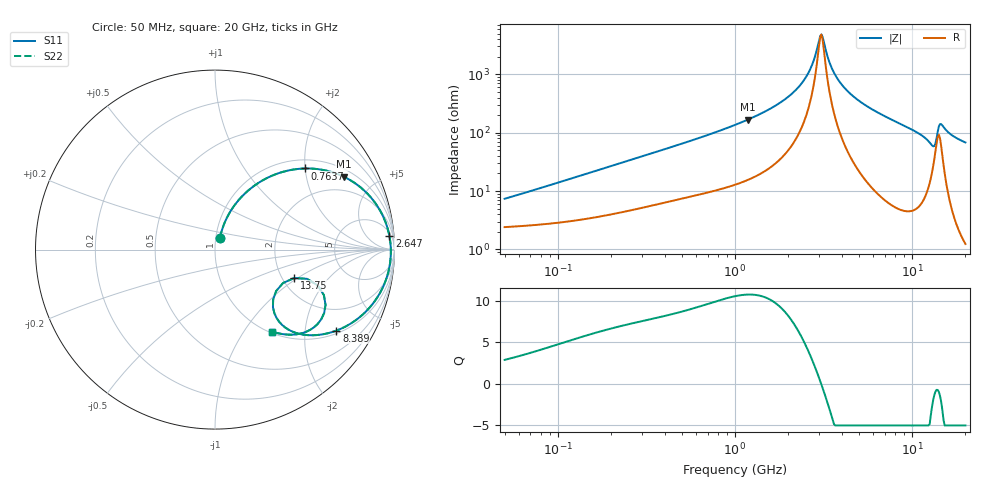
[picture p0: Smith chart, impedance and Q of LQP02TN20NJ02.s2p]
!Murata Part Number: LQP02TN20NJ02
!These Parameters are Measured in Series Mode Connection
!  o--[Z]--o
!Port1  Port2
!  o-------o
!Freq. Start=50[MHz] Stop=20[GHz], 401[Steps]
# Hz S RI R 50
!Freq.(Hz) S11(Real) S11(Imag) S21(Real) S21(Imag) S12(Real) S12(Imag) S22(Real) S22(Imag)
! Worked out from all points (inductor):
!   401 points, 50 MHz to 20 GHz, reference 50 ohm
!   read as one part in series: L = 22 nH near 53.09 MHz
!   highest Q = 10.7 at 1.179 GHz (marker M1), where L = 22.4 nH
!   self-resonance near 3.03 GHz
!   S11 on the Smith chart (normalised r, x): 50 MHz: 1.05, +0.14; 763.7 MHz: 1.20, +1.99; 2.647 GHz: 7, +23; 8.389 GHz: 1.10, -2.93; 13.75 GHz: 2.31, -0.94; 20 GHz: 1.02, -1.36
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5e7  0.028 0.0661  0.972 -0.0661  0.972 -0.0661  0.028 0.0661
1.364002e8  0.0612 0.1672  0.9388 -0.1672  0.9388 -0.1672  0.0612 0.1672
3.721004e8  0.218 0.3552  0.782 -0.3552  0.782 -0.3552  0.218 0.3552
7.636728e8  0.5001 0.4519  0.4999 -0.4519  0.4999 -0.4519  0.5001 0.4519
1e9  0.6362 0.4361  0.3638 -0.4361  0.3638 -0.4361  0.6362 0.4361
1.179116e9  0.7181 0.4058  0.2819 -0.4058  0.2819 -0.4058  0.7181 0.4058
1.99176e9  0.9202 0.2169  0.0798 -0.2169  0.0798 -0.2169  0.9202 0.2169
2.348516e9  0.9556 0.1376  0.0444 -0.1376  0.0444 -0.1376  0.9556 0.1376
2.647493e9  0.9715 0.0768  0.0285 -0.0768  0.0285 -0.0768  0.9715 0.0768
2.728004e9  0.9742 0.0613  0.0258 -0.0613  0.0258 -0.0613  0.9742 0.0613
3.075291e9  0.9797 -0.00135  0.0203 0.00135  0.0203 0.00135  0.9797 -0.00135
3.519108e9  0.9757 -0.0725  0.0243 0.0725  0.0243 0.0725  0.9757 -0.0725
4.087748e9  0.9583 -0.1511  0.0417 0.1511  0.0417 0.1511  0.9583 -0.1511
5.194772e9  0.9012 -0.2712  0.0988 0.2712  0.0988 0.2712  0.9012 -0.2712
7.442007e9  0.7463 -0.4181  0.2537 0.4181  0.2537 0.4181  0.7463 -0.4181
8.389408e9  0.6765 -0.4513  0.3235 0.4513  0.3235 0.4513  0.6765 -0.4513
1.166392e10  0.4226 -0.4528  0.5774 0.4528  0.5774 0.4528  0.4226 -0.4528
1.295331e10  0.3229 -0.3208  0.6771 0.3208  0.6771 0.3208  0.3229 -0.3208
1.375312e10  0.4407 -0.1585  0.5593 0.1585  0.5593 0.1585  0.4407 -0.1585
1.482269e10  0.608 -0.354  0.392 0.354  0.392 0.354  0.608 -0.354
1.621653e10  0.4909 -0.464  0.5091 0.464  0.5091 0.464  0.4909 -0.464
2e10  0.3192 -0.4571  0.6808 0.4571  0.6808 0.4571  0.3192 -0.4571
